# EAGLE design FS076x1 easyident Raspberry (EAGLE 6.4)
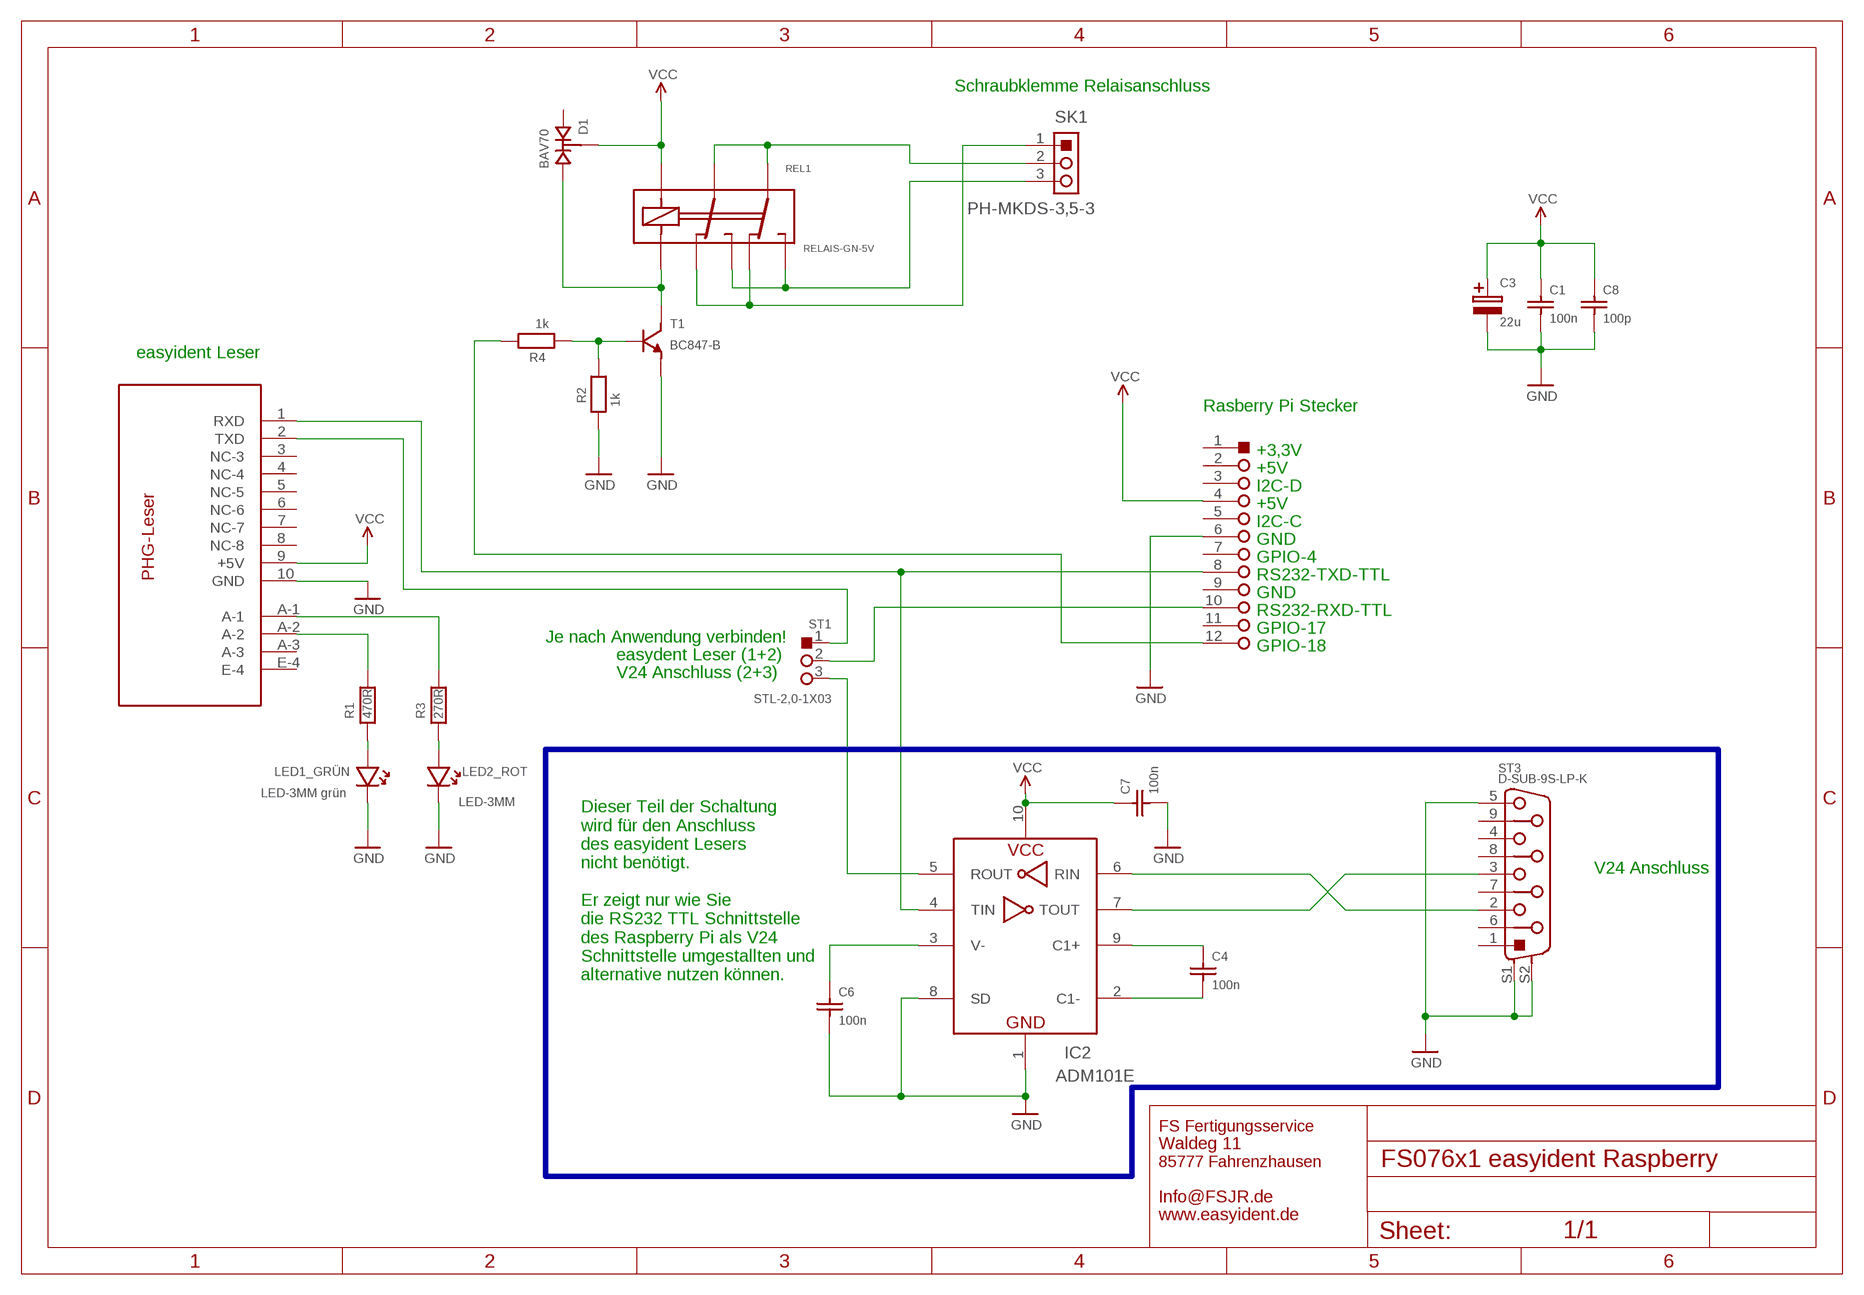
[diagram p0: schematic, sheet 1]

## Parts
C1  100n  C-0603  [0603]
C3  22u  C-TAJA  [TAJA]
C4  100n  C-0603  [0603]
C6  100n  C-0603  [0603]
C7  100n  C-0603  [0603]
C8  100p  C-0603  [0603]
D1  BAV70  [SOT-23]
IC2  ADM101E  [µSOIC-10]
LED1_GRÜN  LED-3MM grün  LED-3MM  [LED-3MM]
LED2_ROT  LED-3MM  [LED-3MM]
MODUL1  PHG-LESER  [PHG-LESER]
R1  470R  R-0603  [0603]
R2  1k  R-0603  [0603]
R3  270R  R-0603  [0603]
R4  1k  R-0603  [0603]
REL1  RELAIS-GN-5V  [RELAIS-GN]
SK1  PH-MKDS-3,5-3  [PH-MKDS-3,5-3]
ST1  STL-2,0-1X03  [STL-2,0-1X03]
ST3  D-SUB-9S-LP-K  [D_SUB-9-STIFT]
ST4  STL-2R-2,54-12  [STL-2R-2,54-12]
T1  BC847-B  [SOT-23]

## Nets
GND: C1.2 C3.M-(-) C6.2 C7.2 C8.2 IC2.1(GND) IC2.8(SD) LED1_GRÜN.K LED2_ROT.K MODUL1.10(GND) R2.2 ST3.5 ST3.S1 ST3.S2 ST4.6 T1.2(E)
LED-GRÜN: MODUL1.A-2 R1.1
LED-ROT: MODUL1.A-1 R3.1
N$1: ST1.2 ST4.10
N$2: MODUL1.2(TXD) ST1.1
N$3: LED1_GRÜN.A R1.2
N$4: LED2_ROT.A R3.2
N$5: C6.1 IC2.3(V-)
N$6: IC2.5(ROUT) ST1.3
N$7: IC2.6(RIN) ST3.2
N$8: C4.1 IC2.9(C1+)
N$9: IC2.7(TOUT) ST3.3
N$10: REL1.3(C1) REL1.6(C2) SK1.2
N$11: C4.2 IC2.2(C1-)
N$12: D1.1 REL1.8(SP-) T1.3(C)
N$13: R2.1 R4.2 T1.1(B)
N$14: R4.1 ST4.12
N$15: REL1.4(NO1) REL1.5(NO2) SK1.3
N$16: REL1.2(NC1) REL1.7(NC2) SK1.1
RXD2_TTL: IC2.4(TIN) MODUL1.1(RXD) ST4.8
VCC: C1.1 C3.P+(+) C7.1 C8.1 D1.3 IC2.10(VCC) MODUL1.9(+5V) REL1.1(SP+) ST4.4
Unconnected: D1.2 MODUL1.3(NC-3) MODUL1.4(NC-4) MODUL1.5(NC-5) MODUL1.6(NC-6) MODUL1.7(NC-7) MODUL1.8(NC-8) MODUL1.A-3 MODUL1.E-4 ST3.1 ST3.4 ST3.6 ST3.7 ST3.8 ST3.9 ST4.1 ST4.2 ST4.3 ST4.5 ST4.7 ST4.9 ST4.11

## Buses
B$1

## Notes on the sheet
- Schraubklemme Relaisanschluss
- easyident Leser
- Rasberry Pi Stecker
- +3,3V
- +5V
- I2C-D
- +5V
- I2C-C
- GND
- GPIO-4
- RS232-TXD-TTL
- GND
- RS232-RXD-TTL
- GPIO-17
- Je nach Anwendung verbinden!
- GPIO-18
- easydent Leser (1+2)
- V24 Anschluss (2+3)
- V24 Anschluss
- Dieser Teil der Schaltung
  wird für den Anschluss 
  des easyident Lesers
  nicht benötigt.
  
  Er zeigt nur wie Sie
  die RS232 TTL Schnittstelle
  des Raspberry Pi als V24 
  Schnittstelle umgestallten und
  alternative nutzen können.

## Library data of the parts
C1 C4 C6-C8 = 5-FS-Library:C-0603
C3 = 5-FS-Kondensatoren:C-TAJA
D1 = 5-FS-Library:BAV70
IC2 = 5-FS-Library:ADM101E
LED1_GRÜN LED2_ROT = 5-FS-Library:LED-3MM
MODUL1 = 5-FS-Library:PHG-LESER
R1-R4 = 5-FS-Library:R-0603: SMD Widerstand Bauform 0603
REL1 = 5-FS-Library:RELAIS-GN-5V
SK1 = 5-FS-Library:PH-MKDS-3,5-3
ST1 = 5-FS-Stecker:STL-2,0-1X03
ST3 = 5-FS-Stecker:D-SUB-9S-LP-K
ST4 = 5-FS-Stecker:STL-2R-2,54-12
T1 = 5-FS-Library:BC847-B

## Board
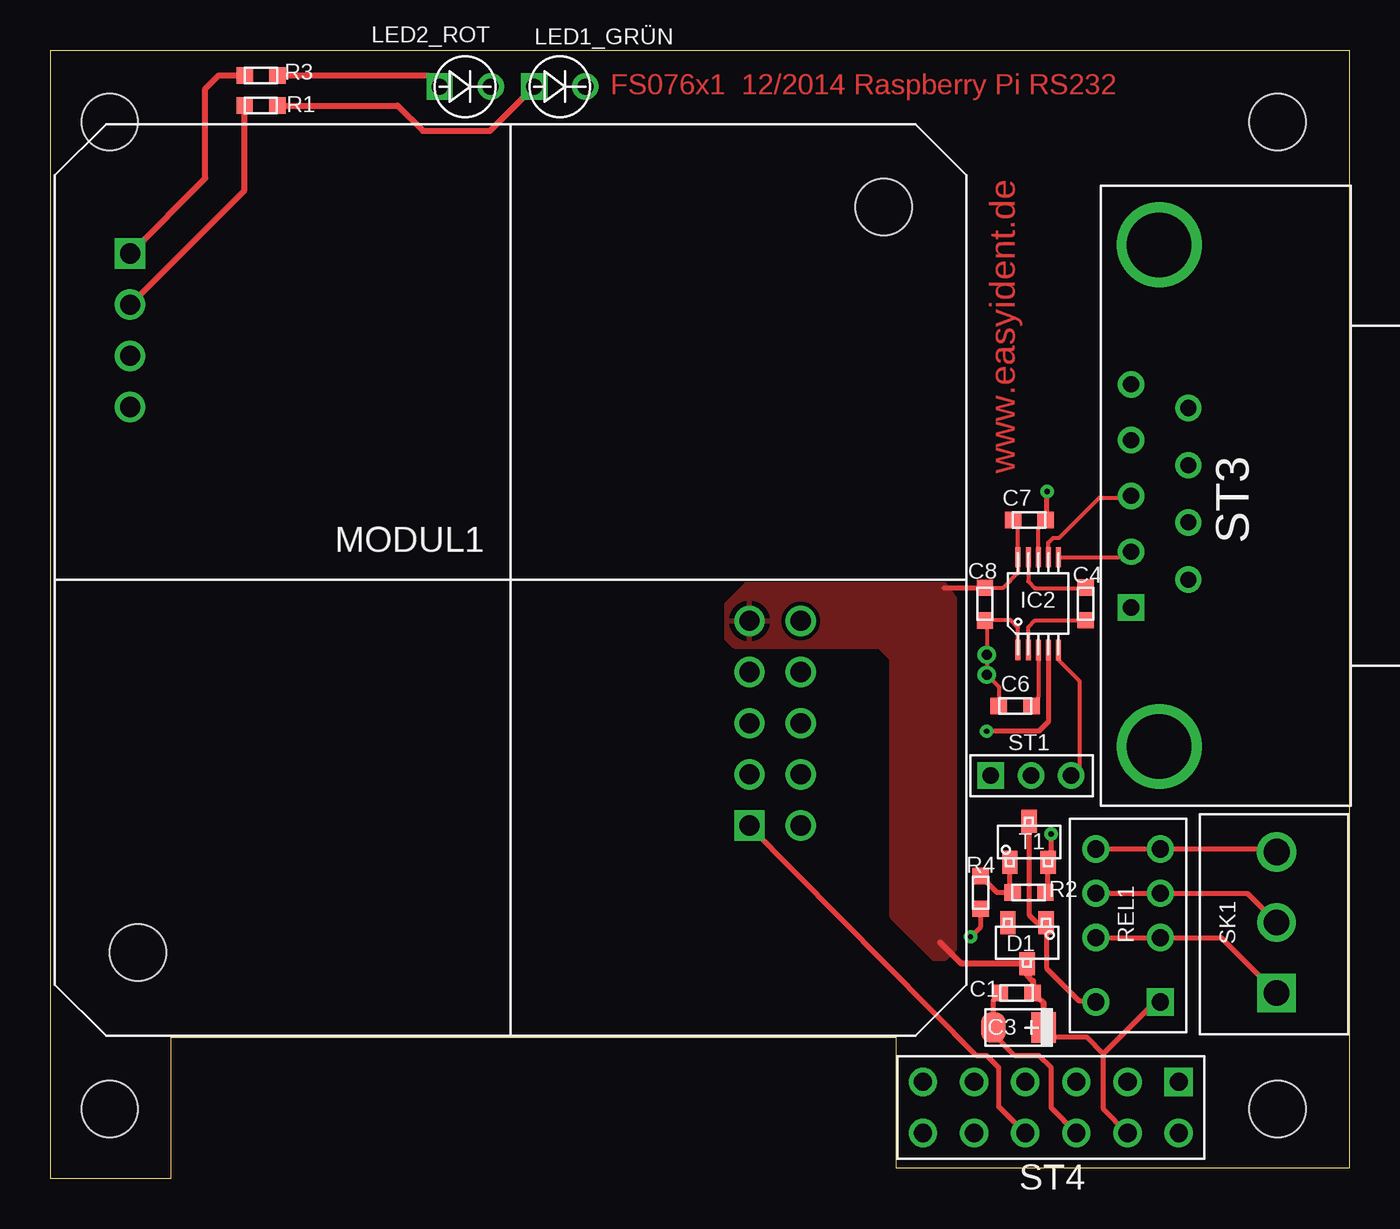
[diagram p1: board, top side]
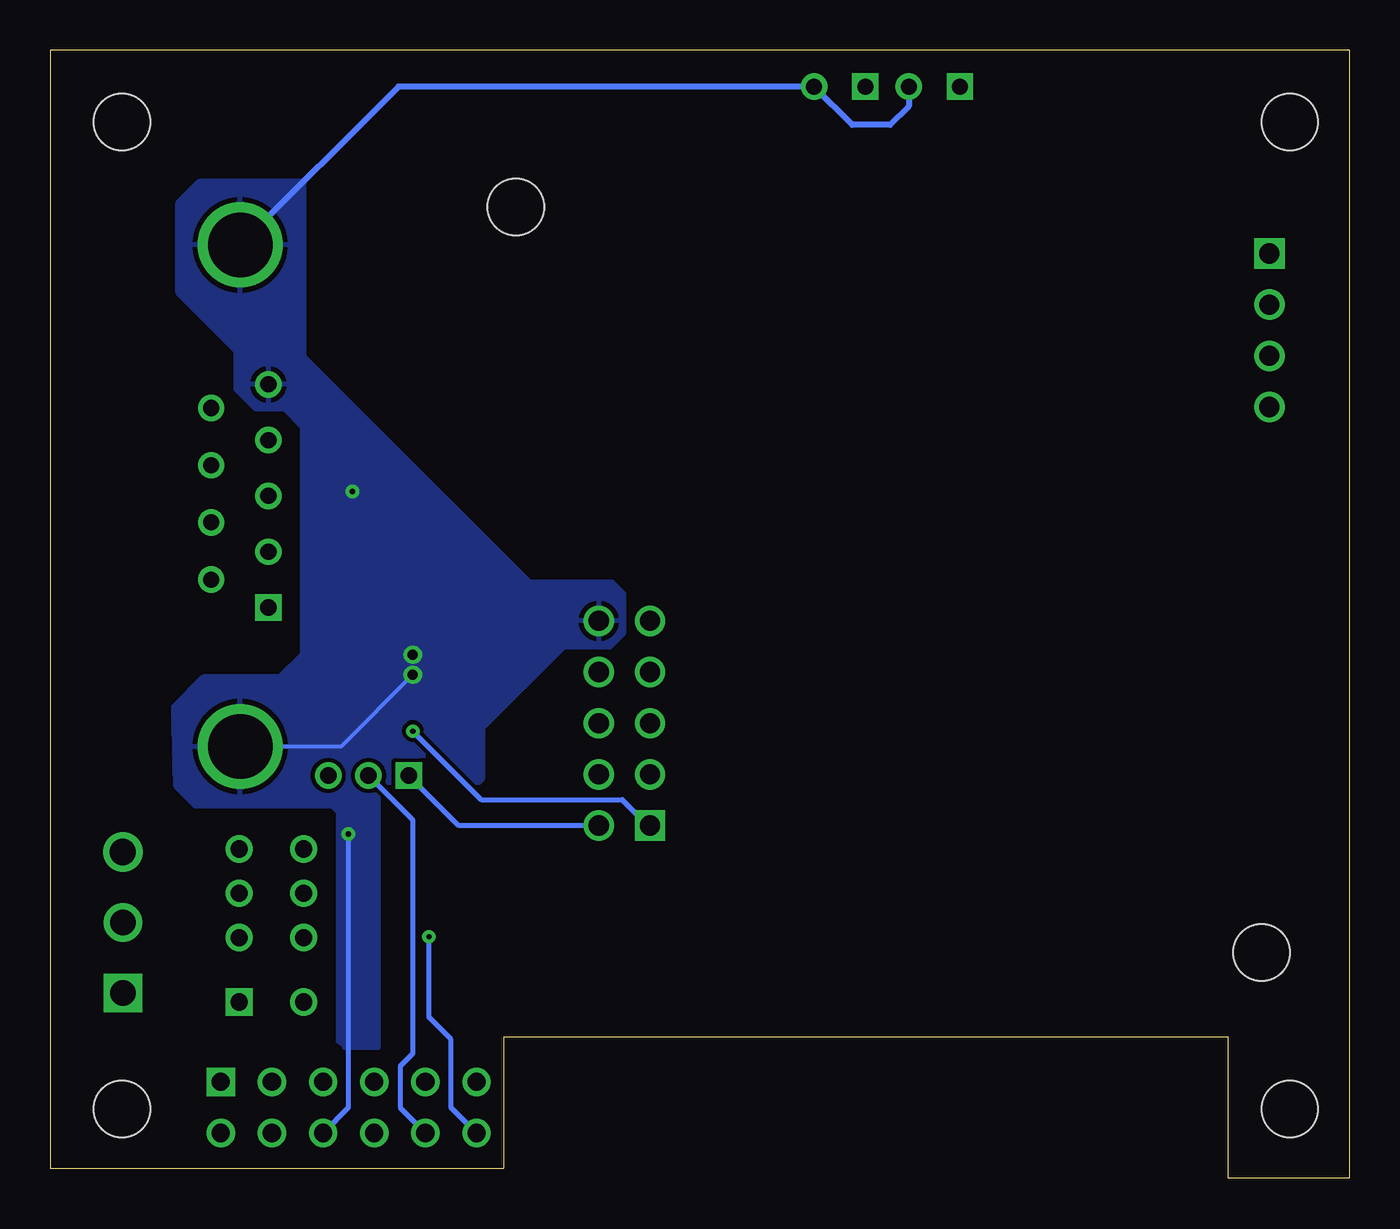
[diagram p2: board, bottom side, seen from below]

Size 64.5 x 56 mm. Coordinates in mm from the lower left corner, seen from the top.
Outline: 0,56 64.5,56 64.5,0.5 42,0.5 42,7 6,7 6,0 0,0 0,56
Copper layers (1*16): Top 0.035mm / dielectric 1.5mm / Bottom 0.035mm
Design rules "default": minimum track width 10mil, minimum drill 24mil, track to track 8mil, track to pad 8mil, pad to pad 8mil, via to via 8mil, smd to smd 8mil, copper to edge 40mil, drill to drill 8mil, minimum pad ring 10mil, minimum via ring 8mil, stop-mask expansion 4mil, vias tented up to drill 0mil, thermal gap 10mil
Holes 2.8 mm at 60.95,3.45 60.95,52.45 2.95,52.45 2.95,3.45

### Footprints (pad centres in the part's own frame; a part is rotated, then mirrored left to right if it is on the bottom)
0603 = smd 0.813 x 0.813: 1 0,0.813; 2 0,-0.813
TAJA = smd 1.2 x 1.5: M- 1.2,0; P+ -1.3,0
SOT-23 = smd 0.762 x 1.143: 1 -0.95,-1; 2 0.95,-1; 3 0,1.032
µSOIC-10 = smd 0.25 x 1: 1 -1,-2.3; 2 -0.5,-2.3; 3 0,-2.3; 4 0.5,-2.3; 5 1,-2.3; 6 1,2.3; 7 0.5,2.3; 8 0,2.3; 9 -0.5,2.3; 10 -1,2.3
LED-3MM = drill 0.8 square: A -1.27,0 | drill 0.8: K 1.27,0
PHG-LESER = drill 1 square: 1 11.862,-12.192; A-1 -18.898,16.205 | drill 1: 2 14.402,-12.192; 3 11.862,-9.652; 4 14.402,-9.652; 5 11.862,-7.112; 6 14.402,-7.112; 7 11.862,-4.572; 8 14.402,-4.572; 9 11.862,-2.032; 10 14.402,-2.032; A-2 -18.898,13.665; A-3 -18.898,11.125; E-4 -18.898,8.585 | hole 2.8: 18.517,18.517; -18.517,-18.491
RELAIS-GN = drill 0.85 square: 1 -4.044,-1.524 | drill 0.85: 2 -0.844,-1.524; 3 1.356,-1.524; 4 3.556,-1.524; 5 3.556,1.676; 6 1.356,1.676; 7 -0.844,1.676; 8 -4.044,1.676
PH-MKDS-3,5-3 = drill 1.27 square: 1 0,0 | drill 1.27: 2 3.5,0 | drill 1.3: 3 7,0
STL-2,0-1X03 = drill 0.813 square: 1 0,0 | drill 0.813: 2 2,0; 3 4,0
D_SUB-9-STIFT = drill 0.8 square: 1 0,0 | drill 0.8: 2 2.77,0; 3 5.54,0; 4 8.31,0; 5 11.08,0; 6 1.385,-2.84; 7 4.225,-2.84; 8 7.065,-2.84; 9 9.905,-2.84 | drill 3.2: S1 -6.9,-1.4; S2 18,-1.4
STL-2R-2,54-12 = drill 0.9 square: 1 0,0 | drill 0.9: 2 0,2.54; 3 2.54,0; 4 2.54,2.54; 5 5.08,0; 6 5.08,2.54; 7 7.62,0; 8 7.62,2.54; 9 10.16,0; 10 10.16,2.54; 11 12.7,0; 12 12.7,2.54

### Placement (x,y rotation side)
C1  47.97,9.21 270 top
C3  48.03,7.49 180 top
C4  51.41,28.52 0 top
C6  47.91,23.46 270 top
C7  48.62,32.69 90 top
C8  46.41,28.51 0 top
D1  48.5,11.7 180 top
IC2  49.06,28.53 0 top
LED1_GRÜN  25.3,54.2 0 top
LED2_ROT  20.6,54.2 0 top
MODUL1  22.86,29.71 0 top
R1  10.46,53.26 90 top
R2  48.6,14.2 90 top
R3  10.47,54.76 90 top
R4  46.2,14.2 180 top
REL1  53.6,12.8 90 top
SK1  60.9,9.2 90 top
ST1  46.7,20 0 top
ST3  53.67,28.34 90 top
ST4  56.03,4.79 180 top
T1  48.6,16.7 0 top

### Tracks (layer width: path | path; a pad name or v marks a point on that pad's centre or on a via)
GND  (via drill 0.25, 0.5)
  Top 0.2: IC2.8 49.06,32.32 C7.2 | C6.2 47.1,24.4 v46.5,25 v46.5,26 46.5,27.61 C8.2 47.7,27.7 48.06,27.34 IC2.1
  Top 0.254: ST4.6 49.7,3.51 49.7,5.5 49.1,6.1 47.9,6.1 46.83,7.17 C3.M- 46.83,8.81 C1.2 | C7.2 49.5,32.76 v49.5,34.1 | R2.2 49.55,14.34 T1.2 49.7,16.25 v49.7,17.1
  Bottom 0.2: v46.5,25 50.06,21.44 ST3.S1
  Bottom 0.254: v49.7,17.1 49.7,3.51 ST4.6
  Bottom 0.305: LED2_ROT.K 21.87,53.23 22.8,52.3 24.67,52.3 LED1_GRÜN.K 47.21,54.2 ST3.S2
  pour Bottom: 39,26.4 36.7,26.4 36,27.1 36,29 36.6,29.6 40.7,29.6 51.9,40.8 51.9,49.5 57.1,49.5 58.2,48.4 58.2,44 55.3,41.1 55.3,39.2 54.3,38.2 52.9,38.2 52,37.3 52,26 53.1,24.9 56.9,24.9 58.4,23.4 58.3,19.5 57.3,18.5 50.5,18.5 50.2,18.2 50.2,6.8 49.9,6.6 49.9,6.5 48.2,6.5 48.2,19.1 43.8,19.1 43,19.9 43,22.4
LED-GRÜN
  Top 0.305: MODUL1.A-2 9.65,49.06 R1.1
LED-ROT
  Top 0.305: MODUL1.A-1 7.7,49.65 7.7,54.1 8.36,54.76 R3.1
N$1
  Bottom 0.254: ST1.2 46.5,17.8 46.5,6.2 47.1,5.6 47.1,3.48 ST4.10
N$2
  Bottom 0.254: MODUL1.2 44.22,17.52 ST1.1
N$3
  Top 0.305: R1.2 17.24,53.26 18.5,52 21.83,52 LED1_GRÜN.A
N$4
  Top 0.305: R3.2 18.77,54.76 LED2_ROT.A
N$5
  Top 0.2: IC2.3 49.06,23.9 C6.1
N$6
  Top 0.2: IC2.5 50.06,25.74 51.1,24.7 51.1,20.4 ST1.3
N$7
  Top 0.2: IC2.6 53.39,30.83 ST3.2
N$8
  Top 0.2: IC2.9 48.56,29.64 48.9,29.3 51.38,29.3 C4.1
N$9
  Top 0.2: IC2.7 49.56,31.56 49.8,31.8 50.1,31.8 52.1,33.8 53.59,33.8 ST3.3
N$10
  Top 0.254: REL1.6 REL1.3 59.44,14.16 SK1.2
N$11
  Top 0.2: IC2.2 48.56,27.36 48.9,27.7 C4.2
N$12
  Top 0.254: REL1.8 51.92,8.78 51.9,8.8 51.1,8.8 49.5,10.4 49.5,12.55 D1.1 49,12.7 48.6,13.1 T1.3
N$13
  Top 0.254: T1.1 47.65,14.34 R2.1 47.01,14.2 R4.2
N$14  (via drill 0.25)
  Top 0.254: v45.7,12 46.2,12.5 R4.1
  Bottom 0.254: ST4.12 44.6,3.52 44.6,6.9 45.7,8 v45.7,12
N$15
  Top 0.254: REL1.5 REL1.4 60.74,16.36 SK1.3
N$16
  Top 0.254: REL1.7 REL1.2 58.14,11.96 SK1.1
RXD2_TTL  (via drill 0.25)
  Top 0.254: IC2.4 49.56,22.66 49.1,22.2 v46.5,22.2 | ST4.8 47.1,3.57 47.1,5.5 46.5,6.1 46,6.1 34.72,17.48 MODUL1.1
  Bottom 0.254: v46.5,22.2 43.1,18.8 36.1,18.8 34.82,17.52 MODUL1.1
VCC
  Top 0.2: 47.8,32.7 C7.1 48.06,32.44 IC2.10 48.06,30.06 47.3,29.3 46.43,29.3 C8.1
  Top 0.254: ST4.4 52.3,3.45 52.3,6.2 | 52.3,6.2 54.86,8.76 REL1.1 | 52.3,6.2 51.5,7 49.7,7 49.33,7.37 C3.P+ | 46.43,29.3 44.4,29.3 | 48.8,9.23 C1.1
  Top 0.305: C3.P+ 49.33,8.71 C1.1 | 44.2,11.7 45.23,10.67 D1.3 48.5,10.1 48.8,9.8 48.8,9.23
  pour Top: 33.6,28.5 34.6,29.5 44.4,29.5 44.9,28.8 44.9,11.4 44.4,10.9 43.9,10.9 41.8,13 41.8,25.8 41.2,26.4 34,26.4 33.6,26.8

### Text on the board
Top: FS076x1 12/2014 Raspberry Pi RS232 | www.easyident.de | Größe: 64,5 x 55,5 mm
